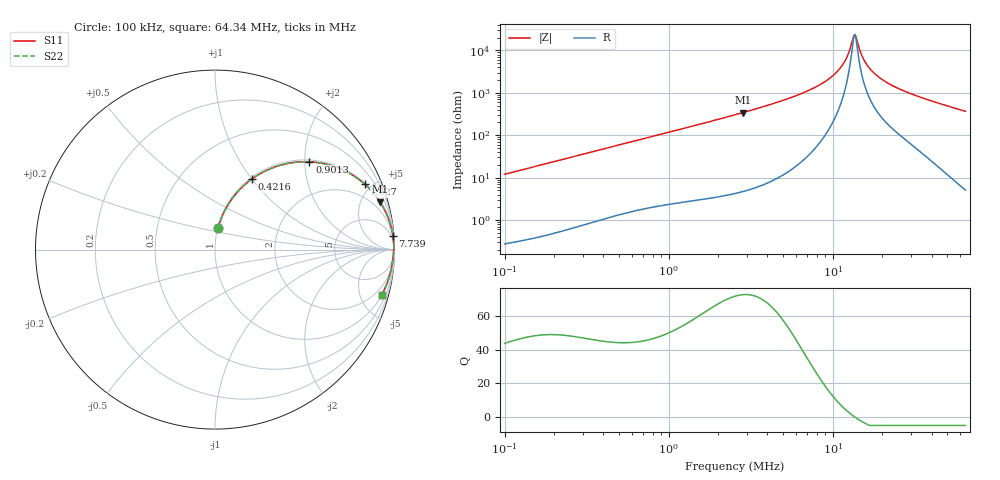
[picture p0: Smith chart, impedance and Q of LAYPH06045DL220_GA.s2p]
! LAYPH06045DL220_GA  S-PARAMETER MODEL  ( General Type )
! Model Generated by TAIYO YUDEN Corporation (http://www.ty-top.com)
! Version 2.0
! TAIYO YUDEN Control No. 180914NI43SB-FBB
! Copyright(c) 2018 TAIYO YUDEN CO.,LTD. All Rights Reserved.
! Product Description (link to TY-COMPAS)
! https://ds.yuden.co.jp/TYCOMPAS/or/detail?pn=LAYPH06045DL220MGA&u=M
! Products Name : Inductors
! Characteristics :
!  Inductance : 22 uH , SRF(min) : -Hz , DC Resistance(max) : 0.0948 Ohm
!  Rated Current : Saturation :1.3 A , Temp Rise : 1.1 A (25 degC)
!  Case Size : 6.3 x 6.0 / 0.248 x 0.236 [mm/inch] , Thickness : 4.5 / 0.177 [mm/inch]
!  (Conditions: Temperature = 25 degC , DC Bias Current/Voltage = 0A / 0V)
! External Node Assignments :
!  1  o---GGG---o  2
! GND o---------o GND
! Frequency Range : 0.1MHz  -  64.339822MHz  [ 402 STEP ]
# MHz S RI R 50
! Freq[MHz].  S11 Real  S11 Imag  S21 Real  S21 Imag  S12 Real  S12 Imag  S22 Real  S22 Imag
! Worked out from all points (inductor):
!   401 points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, 100 kHz to 64.34 MHz, reference 50 ohm
!   read as one part in series: L = 19 uH near 103.3 kHz
!   highest Q = 72.8 at 2.84 MHz (marker M1), where L = 19.2 uH
!   self-resonance near 13.41 MHz
!   S11 on the Smith chart (normalised r, x): 100 kHz: 1.01, +0.24; 421.6 kHz: 1.02, +1.00; 901.3 kHz: 1.04, +2.11; 1.927 MHz: 1.07, +4.55; 7.739 MHz: 2, +26; 64.34 MHz: 1.10, -7.35
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0.1  0.0168 0.1176  0.9832 -0.1176  0.9832 -0.1176  0.0168 0.1176
0.295407  0.1148 0.3083  0.8852 -0.3083  0.8852 -0.3083  0.1148 0.3083
0.421587  0.2043 0.3922  0.7957 -0.3922  0.7957 -0.3922  0.2043 0.3922
0.872651  0.5106 0.4895  0.4894 -0.4895  0.4894 -0.4895  0.5106 0.4895
0.901329  0.5263 0.4891  0.4737 -0.4891  0.4737 -0.4891  0.5263 0.4891
1.92699  0.8342 0.3644  0.1658 -0.3644  0.1658 -0.3644  0.8342 0.3644
2.53653  0.8988 0.2947  0.1012 -0.2947  0.1012 -0.2947  0.8988 0.2947
2.840458  0.9186 0.2667  0.0814 -0.2667  0.0814 -0.2667  0.9186 0.2667
7.493079  0.991 0.0793  0.009 -0.0793  0.009 -0.0793  0.991 0.0793
7.739318  0.9917 0.0746  0.00829 -0.0746  0.00829 -0.0746  0.9917 0.0746
9.549449  0.9949 0.0453  0.00511 -0.0453  0.00511 -0.0453  0.9949 0.0453
11.04509  0.9959 0.0263  0.00413 -0.0263  0.00413 -0.0263  0.9959 0.0263
11.97499  0.996 0.0161  0.00395 -0.0161  0.00395 -0.0161  0.996 0.0161
13.19478  0.9959 0.00394  0.00407 -0.00394  0.00407 -0.00394  0.9959 0.00394
13.62839  0.9958 -6.42e-05  0.00419 6.42e-05  0.00419 6.42e-05  0.9958 -6.42e-05
14.07625  0.9957 -0.00406  0.00434 0.00406  0.00434 0.00406  0.9957 -0.00406
15.26136  0.9951 -0.014  0.00488 0.014  0.00488 0.014  0.9951 -0.014
16.54623  0.9944 -0.0239  0.00563 0.0239  0.00563 0.0239  0.9944 -0.0239
18.8308  0.9927 -0.0399  0.00727 0.0399  0.00727 0.0399  0.9927 -0.0399
22.13506  0.99 -0.0604  0.01 0.0604  0.01 0.0604  0.99 -0.0604
33.70015  0.9786 -0.1206  0.0214 0.1206  0.0214 0.1206  0.9786 -0.1206
64.33982  0.9281 -0.2515  0.0719 0.2515  0.0719 0.2515  0.9281 -0.2515
